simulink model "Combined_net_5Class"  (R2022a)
settings: Solver=FixedStepAuto  StartTime=0.0  StopTime=simtime  FixedStep=1  RelTol=1e-3
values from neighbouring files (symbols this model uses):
  simtime = length(SOC_CC{1, 1})    [Data_preparation.m]    (also in SimulationCycle.m = cell2mat(simtime_og(i)))
  SOH_predict = double(ans.SOHout(simtime))    [SimulationCycle.m]
undefined symbols (not defined in the file or in its folder): dSOC_mu_CC, dSOC_sig_CC, dv_mu_CC, dv_sig_CC, SOC_mu_CC, SOC_sig_CC, SOE_mu_CC, SOE_sig_CC
libraries: neural x183, deeplib x1
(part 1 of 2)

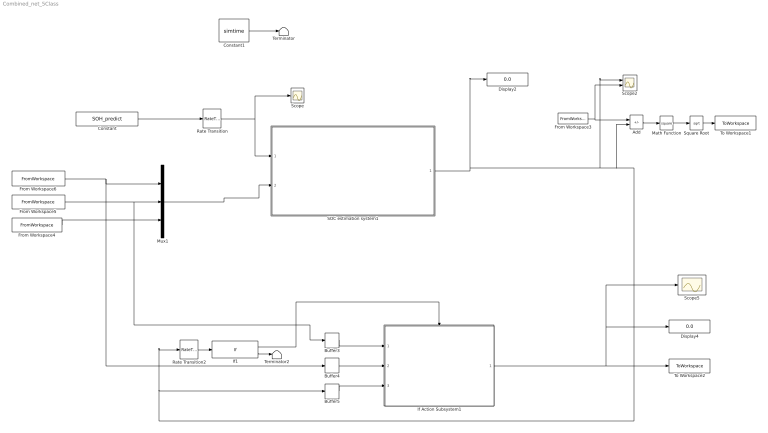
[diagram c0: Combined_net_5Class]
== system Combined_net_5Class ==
  Add : Sum  Inputs=+-
  Buffer3 : Buffer  N=120  OutputFrames=off
  Buffer4 : Buffer  N=120  OutputFrames=off
  Buffer5 : Buffer  N=120  OutputFrames=off
  Constant : Constant  Value=SOH_predict
  Constant1 : Constant  Value=simtime
  Display2 : Display
  Display4 : Display
  From Workspace3 : FromWorkspace  VariableName=SOC_GT
  From Workspace4 : FromWorkspace  VariableName=Temperature
  From Workspace5 : FromWorkspace  VariableName=Voltage  SampleTime=1
  From Workspace6 : FromWorkspace  VariableName=Current  SampleTime=1
  If Action Subsystem1 : Subsystem  TreatAsAtomicUnit=on
  If1 : If  IfExpression=u1 < 0.6
  Math Function : Math  Operator=square
  Mux1 : Mux  Inputs=3
  Rate Transition : RateTransition  OutPortSampleTime=1
  Rate Transition2 : RateTransition  OutPortSampleTime=1
  SOC estimation system1 : Subsystem
  Scope : Scope
  Scope2 : Scope  NumInputPorts=2
  Scope5 : Scope
  Square Root : Sqrt
  Terminator : Terminator
  Terminator2 : Terminator
  To Workspace1 : ToWorkspace  VariableName=SOC_abserror  SampleTime=-1
  To Workspace2 : ToWorkspace  VariableName=SOHout  SampleTime=-1
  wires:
  Rate Transition/1 -> Scope/1, SOC estimation system1/1(SOH)
  Buffer4/1 -> If Action Subsystem1/2(I)
  Buffer5/1 -> If Action Subsystem1/3(SOC)
  From Workspace6/1 -> Mux1/1, Buffer4/1
  Buffer3/1 -> If Action Subsystem1/1(V)
  From Workspace5/1 -> Buffer3/1, Mux1/2
  If1/1 -> If Action Subsystem1/Action
  If Action Subsystem1/1(Output) -> Scope5/1, Display4/1, To Workspace2/1
  Mux1/1 -> SOC estimation system1/2(Input)
  From Workspace4/1 -> Mux1/3
  If1/2 -> Terminator2/1
  Rate Transition2/1 -> If1/1
  Constant/1 -> Rate Transition/1
  Constant1/1 -> Terminator/1
  Math Function/1 -> Square Root/1
  From Workspace3/1 -> Add/1, Scope2/2
  Add/1 -> Math Function/1
  SOC estimation system1/1(SOC) -> Add/2, Rate Transition2/1, Buffer5/1, Scope2/1, Display2/1
  Square Root/1 -> To Workspace1/1

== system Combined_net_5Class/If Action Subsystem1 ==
  V : Inport
  I : Inport  Port=2
  SOC : Inport  Port=3
  Action Port : ActionPort  ActionPortLabel=if(u1 < 0.6)
  SOH estimation system : Subsystem
  Output : Outport
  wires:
  V/1 -> SOH estimation system/1(V)
  I/1 -> SOH estimation system/2(I)
  SOC/1 -> SOH estimation system/3(SOC)
  SOH estimation system/1(Input1) -> Output/1

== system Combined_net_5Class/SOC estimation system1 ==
  SOH : Inport
  Input : Inport  Port=2
  Class 1 : Subsystem
  Class 2 : Subsystem
  Class 3 : Subsystem
  Class 4 : Subsystem
  Class 5 : Subsystem
  If1 : If  IfExpression=0.96<u1  ElseIfExpressions=0.92<u1&u1<=0.96  ShowElse=off
  If2 : If  IfExpression=0.9<u1&u1<=0.92  ElseIfExpressions=0.87<u1&u1<=0.9  ShowElse=off
  If3 : If  IfExpression=u1<=0.87  ShowElse=off
  Merge1 : Merge  Inputs=5
  SOC : Outport
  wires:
  If3/1 -> Class 5/Action
  If2/2 -> Class 4/Action
  Class 3/1(SOC) -> Merge1/3
  Class 2/1(SOC) -> Merge1/2
  Class 1/1(SOC) -> Merge1/1
  If1/1 -> Class 1/Action
  Class 4/1(SOC) -> Merge1/4
  SOH/1 -> If3/1, If1/1, If2/1
  Class 5/1(SOC) -> Merge1/5
  Merge1/1 -> SOC/1
  If1/2 -> Class 2/Action
  If2/1 -> Class 3/Action
  Input/1 -> Class 1/1(Input), Class 2/1(Input1), Class 3/1(Input2), Class 4/1(Input), Class 5/1(Input)

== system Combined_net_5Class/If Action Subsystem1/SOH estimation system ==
  V : Inport
  I : Inport  Port=2
  SOC : Inport  Port=3
  Subsystem1 : Subsystem
  Subsystem2 : Subsystem
  Input1 : Outport
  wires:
  Subsystem1/4(SOE) -> Subsystem2/4(SOE)
  Subsystem1/1(dSOC) -> Subsystem2/1(dSOC)
  Subsystem1/2(dv) -> Subsystem2/2(dv)
  Subsystem1/3(SOC) -> Subsystem2/3(SOC)
  Subsystem2/1(Input1) -> Input1/1
  V/1 -> Subsystem1/1(V_03)
  I/1 -> Subsystem1/2(I_03)
  SOC/1 -> Subsystem1/3(SOC_03)

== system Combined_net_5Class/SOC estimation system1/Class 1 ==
  Input : Inport
  Action Port : ActionPort  ActionPortLabel=if(0.96<u1)
  Class 1 : Subsystem  mask{pi_input_1_delayed_1=[0.507169576059850246707583210081793367862701416015625;-0.46688362562526375398874733946286141872406005859375;-0.4863168465980416410587849895819090306758880615234375], ai_layer_2_delayed_1=-0.99999475321330122401519702179939486086368560791015625}
      mask prompts: pi_input_1_delayed_1 "Preprocessed initial input 1 state at timestep 0."; ai_layer_2_delayed_1 "Initial layer 2 state at timestep 0."
      mask help: NARX Neural Network
  SOC : Outport
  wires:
  Class 1/1(y) -> SOC/1
  Input/1 -> Class 1/1(x)

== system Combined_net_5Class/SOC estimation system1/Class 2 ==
  Input1 : Inport
  Action Port : ActionPort  ActionPortLabel=elseif(0.92<u1&u1<=0.96)
  Class 2 : Subsystem  mask{pi_input_1_delayed_1=[0.5002372291633718770498262529144994914531707763671875;-0.5901898734177215555263273927266709506511688232421875;-0.746840148698884487288296440965496003627777099609375], ai_layer_2_delayed_1=-0.99999334769130043820695163958589546382427215576171875}
      mask prompts: pi_input_1_delayed_1 "Preprocessed initial input 1 state at timestep 0."; ai_layer_2_delayed_1 "Initial layer 2 state at timestep 0."
      mask help: NARX Neural Network
  SOC : Outport
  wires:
  Input1/1 -> Class 2/1(x)
  Class 2/1(y) -> SOC/1

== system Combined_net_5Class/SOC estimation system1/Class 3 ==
  Input2 : Inport
  Action Port : ActionPort  ActionPortLabel=if(0.9<u1&u1<=0.92)
  Class 3 : Subsystem  mask{pi_input_1_delayed_1=[0.5070045647725482940160190992173738777637481689453125;-0.611404153034653230491812792024575173854827880859375;-1.455812101910827660589120569056831300258636474609375], ai_layer_2_delayed_1=-0.99999384932865742481311599476612173020839691162109375}
      mask prompts: pi_input_1_delayed_1 "Preprocessed initial input 1 state at timestep 0."; ai_layer_2_delayed_1 "Initial layer 2 state at timestep 0."
      mask help: NARX Neural Network
  SOC : Outport
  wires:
  Class 3/1(y) -> SOC/1
  Input2/1 -> Class 3/1(x)

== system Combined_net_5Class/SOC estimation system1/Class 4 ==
  Input : Inport
  Action Port : ActionPort  ActionPortLabel=elseif(0.87<u1&u1<=0.9)
  Class 4 : Subsystem  mask{pi_input_1_delayed_1=[0.5133640552995391015400628020870499312877655029296875;-0.60258438818565451811082311905920505523681640625;-0.865604575163398504145106926443986594676971435546875], ai_layer_2_delayed_1=-0.99999156111467002450154950565774925053119659423828125}
      mask prompts: pi_input_1_delayed_1 "Preprocessed initial input 1 state at timestep 0."; ai_layer_2_delayed_1 "Initial layer 2 state at timestep 0."
      mask help: NARX Neural Network
  SOC : Outport
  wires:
  Class 4/1(y) -> SOC/1
  Input/1 -> Class 4/1(x)

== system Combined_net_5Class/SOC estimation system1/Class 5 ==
  Input : Inport
  Action Port : ActionPort  ActionPortLabel=if(u1<=0.87)
  Class 5 : Subsystem  mask{pi_input_1_delayed_1=[0.521325559987726006028196934494189918041229248046875;-0.590428999869605064532152027823030948638916015625;-0.49791819740386955572830629535019397735595703125], ai_layer_2_delayed_1=-0.9999922448082632087107413099147379398345947265625}
      mask prompts: pi_input_1_delayed_1 "Preprocessed initial input 1 state at timestep 0."; ai_layer_2_delayed_1 "Initial layer 2 state at timestep 0."
      mask help: NARX Neural Network
  SOC : Outport
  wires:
  Class 5/1(y) -> SOC/1
  Input/1 -> Class 5/1(x)

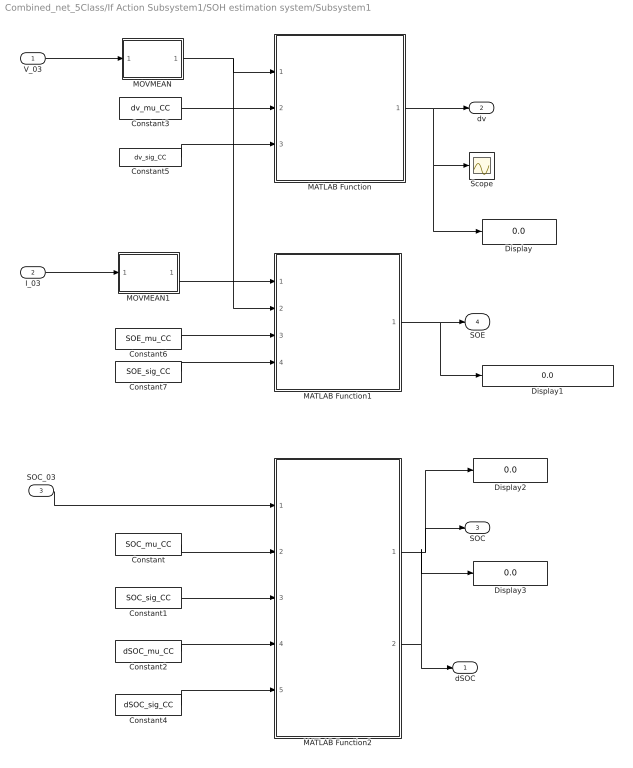
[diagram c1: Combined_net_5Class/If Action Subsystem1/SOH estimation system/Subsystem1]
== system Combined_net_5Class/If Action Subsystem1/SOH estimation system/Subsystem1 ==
  V_03 : Inport
  I_03 : Inport  Port=2
  SOC_03 : Inport  Port=3
  Constant : Constant  Value=SOC_mu_CC
  Constant1 : Constant  Value=SOC_sig_CC
  Constant2 : Constant  Value=dSOC_mu_CC
  Constant3 : Constant  Value=dv_mu_CC
  Constant4 : Constant  Value=dSOC_sig_CC
  Constant5 : Constant  Value=dv_sig_CC
  Constant6 : Constant  Value=SOE_mu_CC
  Constant7 : Constant  Value=SOE_sig_CC
  Display{,1..3} (4 alike) : Display
  MATLAB Function : MATLAB Function  TreatAsAtomicUnit=on
  MATLAB Function1 : MATLAB Function  TreatAsAtomicUnit=on
  MATLAB Function2 : MATLAB Function  TreatAsAtomicUnit=on
  MOVMEAN : MATLAB Function  TreatAsAtomicUnit=on
  MOVMEAN1 : MATLAB Function  TreatAsAtomicUnit=on
  Scope : Scope
  dSOC : Outport
  dv : Outport  Port=2
  SOC : Outport  Port=3
  SOE : Outport  Port=4
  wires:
  Constant4/1 -> MATLAB Function2/5(dSOC_sig_CC)
  Constant6/1 -> MATLAB Function1/3(SOE_mu_CC)
  Constant7/1 -> MATLAB Function1/4(SOE_sig_CC)
  Constant2/1 -> MATLAB Function2/4(dSOC_mu_CC)
  Constant5/1 -> MATLAB Function/3(dv_sig_CC)
  MATLAB Function2/2(dSOC) -> Display3/1, dSOC/1
  MATLAB Function/1(dV) -> Display/1, Scope/1, dv/1
  MATLAB Function2/1(SOC) -> Display2/1, SOC/1
  Constant3/1 -> MATLAB Function/2(dv_mu_CC)
  V_03/1 -> MOVMEAN/1(V)
  I_03/1 -> MOVMEAN1/1(I)
  Constant1/1 -> MATLAB Function2/3(SOC_sig_CC)
  Constant/1 -> MATLAB Function2/2(SOC_mu_CC)
  MATLAB Function1/1(SOE) -> Display1/1, SOE/1
  MOVMEAN/1(V_filt) -> MATLAB Function/1(V_03), MATLAB Function1/2(V_03)
  MOVMEAN1/1(I_filt) -> MATLAB Function1/1(I_03)
  SOC_03/1 -> MATLAB Function2/1(SOC_03)

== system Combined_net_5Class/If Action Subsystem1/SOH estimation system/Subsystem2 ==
  dSOC : Inport
  dv : Inport  Port=2
  SOC : Inport  Port=3
  SOE : Inport  Port=4
  Display : Display
  Mux2 : Mux
  Pulse Generator : DiscretePulseGenerator  PulseType=Time based  Period=120  PulseWidth=1/120*100  PhaseDelay=119
  Resettable Subsystem : Subsystem  TreatAsAtomicUnit=on
  Scope : Scope
  Input1 : Outport
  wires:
  Mux2/1 -> Display/1, Resettable Subsystem/2(Input1)
  dSOC/1 -> Mux2/1
  dv/1 -> Mux2/2
  SOC/1 -> Mux2/3
  SOE/1 -> Mux2/4
  Pulse Generator/1 -> Resettable Subsystem/1(Input), Resettable Subsystem/Reset, Scope/1
  Resettable Subsystem/1(Out1) -> Input1/1

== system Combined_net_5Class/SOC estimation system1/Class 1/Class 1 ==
  x : Inport  PortDimensions=3  SampleTime=1
  Layer 1 : Subsystem
  Layer 2 : Subsystem
  Process Input 1 : Subsystem
  Process Output 1 : Subsystem
  y : Outport  InitialOutput=0
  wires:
  x/1 -> Process Input 1/1(x)
  Process Output 1/1(y) -> y/1
  Process Input 1/1(p) -> Layer 1/1("p{1}")
  Layer 1/1("a{1}") -> [feedback1]
  [feedback1] -> Layer 2/1("a{1} ")
  Layer 2/1("a{2}") -> [feedback2], Process Output 1/1(a)
  [feedback2] -> Layer 1/2("a{2} ")

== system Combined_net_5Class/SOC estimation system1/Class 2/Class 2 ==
  x : Inport  PortDimensions=3  SampleTime=1
  Layer 1 : Subsystem
  Layer 2 : Subsystem
  Process Input 1 : Subsystem
  Process Output 1 : Subsystem
  y : Outport  InitialOutput=0
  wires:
  x/1 -> Process Input 1/1(x)
  Process Output 1/1(y) -> y/1
  Process Input 1/1(p) -> Layer 1/1("p{1}")
  Layer 1/1("a{1}") -> [feedback1]
  [feedback1] -> Layer 2/1("a{1} ")
  Layer 2/1("a{2}") -> [feedback2], Process Output 1/1(a)
  [feedback2] -> Layer 1/2("a{2} ")

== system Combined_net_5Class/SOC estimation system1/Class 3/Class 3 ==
  x : Inport  PortDimensions=3  SampleTime=1
  Layer 1 : Subsystem
  Layer 2 : Subsystem
  Process Input 1 : Subsystem
  Process Output 1 : Subsystem
  y : Outport  InitialOutput=0
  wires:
  x/1 -> Process Input 1/1(x)
  Process Output 1/1(y) -> y/1
  Process Input 1/1(p) -> Layer 1/1("p{1}")
  Layer 1/1("a{1}") -> [feedback1]
  [feedback1] -> Layer 2/1("a{1} ")
  Layer 2/1("a{2}") -> [feedback2], Process Output 1/1(a)
  [feedback2] -> Layer 1/2("a{2} ")

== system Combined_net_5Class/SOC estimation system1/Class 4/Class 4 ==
  x : Inport  PortDimensions=3  SampleTime=1
  Layer 1 : Subsystem
  Layer 2 : Subsystem
  Process Input 1 : Subsystem
  Process Output 1 : Subsystem
  y : Outport  InitialOutput=0
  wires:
  x/1 -> Process Input 1/1(x)
  Process Output 1/1(y) -> y/1
  Process Input 1/1(p) -> Layer 1/1("p{1}")
  Layer 1/1("a{1}") -> [feedback1]
  [feedback1] -> Layer 2/1("a{1} ")
  Layer 2/1("a{2}") -> [feedback2], Process Output 1/1(a)
  [feedback2] -> Layer 1/2("a{2} ")

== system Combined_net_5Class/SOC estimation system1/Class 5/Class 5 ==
  x : Inport  PortDimensions=3  SampleTime=1
  Layer 1 : Subsystem
  Layer 2 : Subsystem
  Process Input 1 : Subsystem
  Process Output 1 : Subsystem
  y : Outport  InitialOutput=0
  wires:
  x/1 -> Process Input 1/1(x)
  Process Output 1/1(y) -> y/1
  Process Input 1/1(p) -> Layer 1/1("p{1}")
  Layer 1/1("a{1}") -> [feedback1]
  [feedback1] -> Layer 2/1("a{1} ")
  Layer 2/1("a{2}") -> [feedback2], Process Output 1/1(a)
  [feedback2] -> Layer 1/2("a{2} ")

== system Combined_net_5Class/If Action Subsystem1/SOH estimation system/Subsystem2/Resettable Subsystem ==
  Input : Inport
  Input1 : Inport  Port=2
  Reset : ResetPort  DisableCoverage=on
  Triggered Subsystem : Subsystem  TreatAsAtomicUnit=on
  Out1 : Outport
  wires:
  Triggered Subsystem/1(Out1) -> Out1/1
  Input/1 -> Triggered Subsystem/Trigger
  Input1/1 -> Triggered Subsystem/1(u)

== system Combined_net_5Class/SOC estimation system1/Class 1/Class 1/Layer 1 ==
  "p{1}" : Inport  PortDimensions=3  SampleTime=1
  "a{2} " : Inport  Port=2  PortDimensions=1  SampleTime=1
  Delays 1 : Subsystem
  Delays 2 : Subsystem
  "IW{1,1}" : Subsystem
  "LW{1,2}" : Subsystem
  "b{1}" : Constant  Value=[2.34272603015963820638489778502844274044036865234375;-1.83098571478465554918102498049847781658172607421875;-0.79131154125893576889438918442465364933013916015625;-1.2076273263687624659468156096409074962139129638671875;0.84071386902655909079129514793748967349529266357421875;-0.53056878404548457606182410017936490476131439208984375;-0.0240383625943490740473063027593525475822389125823974609375;0.16604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
  netsum : Sum  Inputs=3  InputSameDT=on  SaturateOnIntegerOverflow=on
  tansig : neural/Transfer Functions/tansig
  "a{1}" : Outport  InitialOutput=[0;0;0;0;0;0;0;0;0;0;0;0;0;0;0]
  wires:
  "p{1}"/1 -> Delays 1/1("p{1}")
  Delays 1/1("pd{1,1}") -> "IW{1,1}"/1("pd{1,1}")
  "IW{1,1}"/1("iz{1,1}") -> netsum/1
  "a{2} "/1 -> Delays 2/1("p{1}")
  Delays 2/1("pd{1,2}") -> "LW{1,2}"/1("ad{1,2}")
  "LW{1,2}"/1("lz{1,2}") -> netsum/2
  "b{1}"/1 -> netsum/3
  netsum/1 -> tansig/1
  tansig/1 -> "a{1}"/1

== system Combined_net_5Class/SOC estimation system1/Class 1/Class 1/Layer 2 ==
  "a{1} " : Inport  PortDimensions=15  SampleTime=1
  Delays 1 : Subsystem
  "LW{2,1}" : Subsystem
  "b{2}" : Constant  Value=-0.2610570456976468722842810166184790432453155517578125
  netsum : Sum  Inputs=2  InputSameDT=on  SaturateOnIntegerOverflow=on
  purelin : neural/Transfer Functions/purelin
  "a{2}" : Outport  InitialOutput=0
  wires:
  "a{1} "/1 -> Delays 1/1("p{2}")
  Delays 1/1("pd{2,1}") -> "LW{2,1}"/1("ad{2,1}")
  "LW{2,1}"/1("lz{2,1}") -> netsum/1
  "b{2}"/1 -> netsum/2
  netsum/1 -> purelin/1
  purelin/1 -> "a{2}"/1

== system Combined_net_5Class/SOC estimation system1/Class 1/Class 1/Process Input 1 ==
  x : Inport  PortDimensions=3  SampleTime=1
  mapminmax : neural/Processing Functions/mapminmax  xmin=[-4.82500000000000017763568394003;2.50570000000000003836930773105;17.1380000000000016768808563938]  xmax=[1.5909999999999999698019337302;4.16500000000000003552713678801;25.1039999999999992041921359487]  ymin=-1  ymax=1
  p : Outport  PortDimensions=3  SampleTime=1
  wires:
  x/1 -> mapminmax/1
  mapminmax/1 -> p/1

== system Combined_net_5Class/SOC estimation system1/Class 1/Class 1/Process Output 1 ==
  a : Inport  PortDimensions=1  SampleTime=1
  mapminmax_reverse : neural/Processing Functions/mapminmax_reverse  xmin=-2.62341179120179950748424461959e-06  xmax=1.00000440635255594123975697585  ymin=-1  ymax=1
  y : Outport  PortDimensions=1  SampleTime=1
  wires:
  a/1 -> mapminmax_reverse/1
  mapminmax_reverse/1 -> y/1

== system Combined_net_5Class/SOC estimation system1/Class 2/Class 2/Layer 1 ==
  "p{1}" : Inport  PortDimensions=3  SampleTime=1
  "a{2} " : Inport  Port=2  PortDimensions=1  SampleTime=1
  Delays 1 : Subsystem
  Delays 2 : Subsystem
  "IW{1,1}" : Subsystem
  "LW{1,2}" : Subsystem
  "b{1}" : Constant  Value=[2.123679128509173619221428452874533832073211669921875;-2.87621199885181422217783619998954236507415771484375;-0.54420836494168567387674784185946919023990631103515625;-0.5394065908795988573132262899889610707759857177734375;0.85139936745729760669831875929958187043666839599609375;-1.1563643607811477931335275570745579898357391357421875;-0.61089692546734919442741329476120881736278533935546875;-0.197690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
  netsum : Sum  Inputs=3  InputSameDT=on  SaturateOnIntegerOverflow=on
  tansig : neural/Transfer Functions/tansig
  "a{1}" : Outport  InitialOutput=[0;0;0;0;0;0;0;0;0;0;0;0;0;0;0;0]
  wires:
  "p{1}"/1 -> Delays 1/1("p{1}")
  Delays 1/1("pd{1,1}") -> "IW{1,1}"/1("pd{1,1}")
  "IW{1,1}"/1("iz{1,1}") -> netsum/1
  "a{2} "/1 -> Delays 2/1("p{1}")
  Delays 2/1("pd{1,2}") -> "LW{1,2}"/1("ad{1,2}")
  "LW{1,2}"/1("lz{1,2}") -> netsum/2
  "b{1}"/1 -> netsum/3
  netsum/1 -> tansig/1
  tansig/1 -> "a{1}"/1

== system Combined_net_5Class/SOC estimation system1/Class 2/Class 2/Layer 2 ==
  "a{1} " : Inport  PortDimensions=16  SampleTime=1
  Delays 1 : Subsystem
  "LW{2,1}" : Subsystem
  "b{2}" : Constant  Value=0.1380564376019000061290853409445844590663909912109375
  netsum : Sum  Inputs=2  InputSameDT=on  SaturateOnIntegerOverflow=on
  purelin : neural/Transfer Functions/purelin
  "a{2}" : Outport  InitialOutput=0
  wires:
  "a{1} "/1 -> Delays 1/1("p{2}")
  Delays 1/1("pd{2,1}") -> "LW{2,1}"/1("ad{2,1}")
  "LW{2,1}"/1("lz{2,1}") -> netsum/1
  "b{2}"/1 -> netsum/2
  netsum/1 -> purelin/1
  purelin/1 -> "a{2}"/1

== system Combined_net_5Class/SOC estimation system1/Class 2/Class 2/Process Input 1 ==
  x : Inport  PortDimensions=3  SampleTime=1
  mapminmax : neural/Processing Functions/mapminmax  xmin=[-4.73300000000000054001247917768;2.63719999999999998863131622784;17.8219999999999991757704265183]  xmax=[1.59000000000000007993605777301;4.15399999999999991473487170879;28.5820000000000007389644451905]  ymin=-1  ymax=1
  p : Outport  PortDimensions=3  SampleTime=1
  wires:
  x/1 -> mapminmax/1
  mapminmax/1 -> p/1

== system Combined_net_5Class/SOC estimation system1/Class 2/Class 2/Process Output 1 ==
  a : Inport  PortDimensions=1  SampleTime=1
  mapminmax_reverse : neural/Processing Functions/mapminmax_reverse  xmin=-3.32617917940104848405083806662e-06  xmax=1.00000413879150817919594373961  ymin=-1  ymax=1
  y : Outport  PortDimensions=1  SampleTime=1
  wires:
  a/1 -> mapminmax_reverse/1
  mapminmax_reverse/1 -> y/1

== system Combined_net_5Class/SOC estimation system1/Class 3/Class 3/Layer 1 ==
  "p{1}" : Inport  PortDimensions=3  SampleTime=1
  "a{2} " : Inport  Port=2  PortDimensions=1  SampleTime=1
  Delays 1 : Subsystem
  Delays 2 : Subsystem
  "IW{1,1}" : Subsystem
  "LW{1,2}" : Subsystem
  "b{1}" : Constant  Value=[-1.93346371221756019309623297885991632938385009765625;1.7923652112547914239115698364912532269954681396484375;1.1238522489621971534035083095659501850605010986328125;0.323356733008480279334406759517150931060314178466796875;0.76493308526969572280762577065615914762020111083984375;-0.351089604850296443938617585445172153413295745849609375;0.33583797370279000471526842375169508159160614013671875;-0.46332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
  netsum : Sum  Inputs=3  InputSameDT=on  SaturateOnIntegerOverflow=on
  tansig : neural/Transfer Functions/tansig
  "a{1}" : Outport  InitialOutput=[0;0;0;0;0;0;0;0;0;0;0;0;0;0;0]
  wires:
  "p{1}"/1 -> Delays 1/1("p{1}")
  Delays 1/1("pd{1,1}") -> "IW{1,1}"/1("pd{1,1}")
  "IW{1,1}"/1("iz{1,1}") -> netsum/1
  "a{2} "/1 -> Delays 2/1("p{1}")
  Delays 2/1("pd{1,2}") -> "LW{1,2}"/1("ad{1,2}")
  "LW{1,2}"/1("lz{1,2}") -> netsum/2
  "b{1}"/1 -> netsum/3
  netsum/1 -> tansig/1
  tansig/1 -> "a{1}"/1

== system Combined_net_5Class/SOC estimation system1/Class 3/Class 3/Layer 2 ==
  "a{1} " : Inport  PortDimensions=15  SampleTime=1
  Delays 1 : Subsystem
  "LW{2,1}" : Subsystem
  "b{2}" : Constant  Value=0.272834520121191526076387390276067890226840972900390625
  netsum : Sum  Inputs=2  InputSameDT=on  SaturateOnIntegerOverflow=on
  purelin : neural/Transfer Functions/purelin
  "a{2}" : Outport  InitialOutput=0
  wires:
  "a{1} "/1 -> Delays 1/1("p{2}")
  Delays 1/1("pd{2,1}") -> "LW{2,1}"/1("ad{2,1}")
  "LW{2,1}"/1("lz{2,1}") -> netsum/1
  "b{2}"/1 -> netsum/2
  netsum/1 -> purelin/1
  purelin/1 -> "a{2}"/1

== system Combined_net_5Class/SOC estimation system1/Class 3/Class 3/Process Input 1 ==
  x : Inport  PortDimensions=3  SampleTime=1
  mapminmax : neural/Processing Functions/mapminmax  xmin=[-4.77700000000000013500311979442;2.6570000000000000284217094304;21.4740000000000001989519660128]  xmax=[1.57600000000000006750155989721;4.15470000000000005968558980385;31.5220000000000020179413695587]  ymin=-1  ymax=1
  p : Outport  PortDimensions=3  SampleTime=1
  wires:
  x/1 -> mapminmax/1
  mapminmax/1 -> p/1

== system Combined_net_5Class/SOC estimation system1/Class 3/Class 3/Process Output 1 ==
  a : Inport  PortDimensions=1  SampleTime=1
  mapminmax_reverse : neural/Processing Functions/mapminmax_reverse  xmin=-3.07535918984610110574521267546e-06  xmax=1.00000457212472371182343522378  ymin=-1  ymax=1
  y : Outport  PortDimensions=1  SampleTime=1
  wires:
  a/1 -> mapminmax_reverse/1
  mapminmax_reverse/1 -> y/1

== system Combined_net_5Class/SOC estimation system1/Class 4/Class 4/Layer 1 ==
  "p{1}" : Inport  PortDimensions=3  SampleTime=1
  "a{2} " : Inport  Port=2  PortDimensions=1  SampleTime=1
  Delays 1 : Subsystem
  Delays 2 : Subsystem
  "IW{1,1}" : Subsystem
  "LW{1,2}" : Subsystem
  "b{1}" : Constant  Value=[-2.688444044962437828871770761907100677490234375;0.858381113224772729353162503684870898723602294921875;-2.222715747204785596835563410422764718532562255859375;1.3209762857863693863436083120177499949932098388671875;-0.8915787953875426996575015436974354088306427001953125;-0.88615966223780884281069347707671113312244415283203125;0.280218393721010927688297442728071473538875579833984375;0.21524348971530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
  netsum : Sum  Inputs=3  InputSameDT=on  SaturateOnIntegerOverflow=on
  tansig : neural/Transfer Functions/tansig
  "a{1}" : Outport  InitialOutput=[0;0;0;0;0;0;0;0;0;0;0;0;0;0;0]
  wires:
  "p{1}"/1 -> Delays 1/1("p{1}")
  Delays 1/1("pd{1,1}") -> "IW{1,1}"/1("pd{1,1}")
  "IW{1,1}"/1("iz{1,1}") -> netsum/1
  "a{2} "/1 -> Delays 2/1("p{1}")
  Delays 2/1("pd{1,2}") -> "LW{1,2}"/1("ad{1,2}")
  "LW{1,2}"/1("lz{1,2}") -> netsum/2
  "b{1}"/1 -> netsum/3
  netsum/1 -> tansig/1
  tansig/1 -> "a{1}"/1

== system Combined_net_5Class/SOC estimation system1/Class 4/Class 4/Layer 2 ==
  "a{1} " : Inport  PortDimensions=15  SampleTime=1
  Delays 1 : Subsystem
  "LW{2,1}" : Subsystem
  "b{2}" : Constant  Value=0.045626078950611735629561138694043620489537715911865234375
  netsum : Sum  Inputs=2  InputSameDT=on  SaturateOnIntegerOverflow=on
  purelin : neural/Transfer Functions/purelin
  "a{2}" : Outport  InitialOutput=0
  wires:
  "a{1} "/1 -> Delays 1/1("p{2}")
  Delays 1/1("pd{2,1}") -> "LW{2,1}"/1("ad{2,1}")
  "LW{2,1}"/1("lz{2,1}") -> netsum/1
  "b{2}"/1 -> netsum/2
  netsum/1 -> purelin/1
  purelin/1 -> "a{2}"/1

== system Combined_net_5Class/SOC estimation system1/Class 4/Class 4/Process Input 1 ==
  x : Inport  PortDimensions=3  SampleTime=1
  mapminmax : neural/Processing Functions/mapminmax  xmin=[-4.91600000000000036948222259525;2.64660000000000028563817977556;18.5259999999999998010480339872]  xmax=[1.59400000000000008348877145181;4.16340000000000021174173525651;28.3180000000000013926637620898]  ymin=-1  ymax=1
  p : Outport  PortDimensions=3  SampleTime=1
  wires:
  x/1 -> mapminmax/1
  mapminmax/1 -> p/1

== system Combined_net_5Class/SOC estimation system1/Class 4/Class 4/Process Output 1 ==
  a : Inport  PortDimensions=1  SampleTime=1
  mapminmax_reverse : neural/Processing Functions/mapminmax_reverse  xmin=-4.21949321457851519659313158095e-06  xmax=1.00000776066564278643511443079  ymin=-1  ymax=1
  y : Outport  PortDimensions=1  SampleTime=1
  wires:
  a/1 -> mapminmax_reverse/1
  mapminmax_reverse/1 -> y/1

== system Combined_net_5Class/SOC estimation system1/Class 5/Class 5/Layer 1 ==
  "p{1}" : Inport  PortDimensions=3  SampleTime=1
  "a{2} " : Inport  Port=2  PortDimensions=1  SampleTime=1
  Delays 1 : Subsystem
  Delays 2 : Subsystem
  "IW{1,1}" : Subsystem
  "LW{1,2}" : Subsystem
  "b{1}" : Constant  Value=[-1.9239326886795684590225619103875942528247833251953125;-1.4156259333430829538968964698142372071743011474609375;-1.8809744346361843003734293233719654381275177001953125;-1.106968201899322767900457620271481573581695556640625;1.16695809702027997190043606678955256938934326171875;1.0579085603689832861817876619170419871807098388671875;0.33221840417104486764543480603606440126895904541015625;-0.035398306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
  netsum : Sum  Inputs=3  InputSameDT=on  SaturateOnIntegerOverflow=on
  tansig : neural/Transfer Functions/tansig
  "a{1}" : Outport  InitialOutput=[0;0;0;0;0;0;0;0;0;0;0;0;0;0;0;0;0;0]
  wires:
  "p{1}"/1 -> Delays 1/1("p{1}")
  Delays 1/1("pd{1,1}") -> "IW{1,1}"/1("pd{1,1}")
  "IW{1,1}"/1("iz{1,1}") -> netsum/1
  "a{2} "/1 -> Delays 2/1("p{1}")
  Delays 2/1("pd{1,2}") -> "LW{1,2}"/1("ad{1,2}")
  "LW{1,2}"/1("lz{1,2}") -> netsum/2
  "b{1}"/1 -> netsum/3
  netsum/1 -> tansig/1
  tansig/1 -> "a{1}"/1

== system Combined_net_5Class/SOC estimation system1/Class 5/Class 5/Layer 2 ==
  "a{1} " : Inport  PortDimensions=18  SampleTime=1
  Delays 1 : Subsystem
  "LW{2,1}" : Subsystem
  "b{2}" : Constant  Value=0.2439901834476533026840883167096762917935848236083984375
  netsum : Sum  Inputs=2  InputSameDT=on  SaturateOnIntegerOverflow=on
  purelin : neural/Transfer Functions/purelin
  "a{2}" : Outport  InitialOutput=0
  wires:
  "a{1} "/1 -> Delays 1/1("p{2}")
  Delays 1/1("pd{2,1}") -> "LW{2,1}"/1("ad{2,1}")
  "LW{2,1}"/1("lz{2,1}") -> netsum/1
  "b{2}"/1 -> netsum/2
  netsum/1 -> purelin/1
  purelin/1 -> "a{2}"/1

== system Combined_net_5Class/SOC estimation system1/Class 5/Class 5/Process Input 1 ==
  x : Inport  PortDimensions=3  SampleTime=1
  mapminmax : neural/Processing Functions/mapminmax  xmin=[-4.94800000000000039790393202566;2.6339000000000001300293206441;17.1340000000000003410605131648]  xmax=[1.57000000000000006217248937901;4.16769999999999996020960679743;25.3000000000000007105427357601]  ymin=-1  ymax=1
  p : Outport  PortDimensions=3  SampleTime=1
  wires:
  x/1 -> mapminmax/1
  mapminmax/1 -> p/1

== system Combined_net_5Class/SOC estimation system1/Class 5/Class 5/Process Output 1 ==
  a : Inport  PortDimensions=1  SampleTime=1
  mapminmax_reverse : neural/Processing Functions/mapminmax_reverse  xmin=-3.87764264893447179729721319141e-06  xmax=1.0000081866738852465203990505  ymin=-1  ymax=1
  y : Outport  PortDimensions=1  SampleTime=1
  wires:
  a/1 -> mapminmax_reverse/1
  mapminmax_reverse/1 -> y/1

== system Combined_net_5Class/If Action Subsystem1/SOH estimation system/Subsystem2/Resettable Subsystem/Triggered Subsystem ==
  u : Inport
  Trigger : TriggerPort  TriggerType=falling  VariantControl=(inherit)
  Display : Display
  Scope : Scope
  Stateful Predict : deeplib/Stateful Predict  Network=Network from MAT-file  NetworkFunction=untitled  NetworkFilePath=E:\Thesis\Conclusion step\net.mat  InputDataFormats={ '', '' }  SampleTime=-1  ForceInterpretedSim=off  EnableDLNetwork=on
  Out1 : Outport
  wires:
  u/1 -> Stateful Predict/1, Scope/1, Display/1
  Stateful Predict/1 -> Out1/1

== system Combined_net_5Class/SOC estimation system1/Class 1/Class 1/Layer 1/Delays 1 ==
  "p{1}" : Inport  PortDimensions=3  SampleTime=1
  Delay 1 : UnitDelay  InitialCondition=pi_input_1_delayed_1
  mux : Mux  Inputs=2
  "pd{1,1}" : Outport
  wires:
  "p{1}"/1 -> Delay 1/1, mux/1
  Delay 1/1 -> mux/2
  mux/1 -> "pd{1,1}"/1

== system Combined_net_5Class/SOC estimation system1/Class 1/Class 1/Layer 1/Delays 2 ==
  "p{1}" : Inport  PortDimensions=1  SampleTime=1
  Delay 1 : UnitDelay  InitialCondition=ai_layer_2_delayed_1
  mux : Mux  Inputs=1
  "pd{1,2}" : Outport
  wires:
  "p{1}"/1 -> Delay 1/1
  Delay 1/1 -> mux/1
  mux/1 -> "pd{1,2}"/1

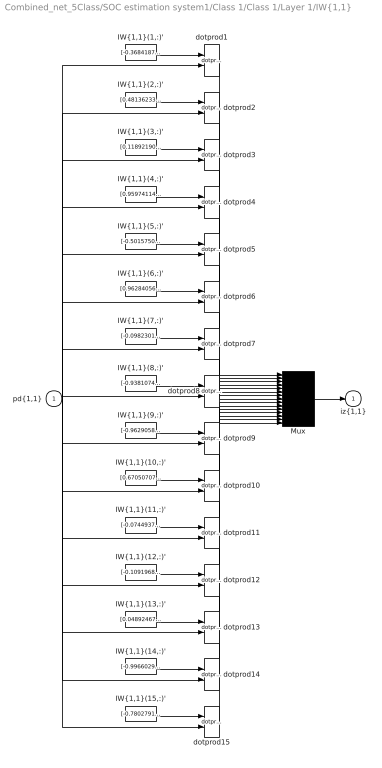
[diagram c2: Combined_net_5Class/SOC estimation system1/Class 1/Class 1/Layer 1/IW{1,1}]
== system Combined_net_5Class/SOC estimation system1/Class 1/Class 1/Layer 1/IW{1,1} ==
  "pd{1,1}" : Inport  PortDimensions=6  SampleTime=1
  "IW{1,1}(1,:)'" : Constant  Value=[-0.36841871672555603911547450479702092707157135009765625;0.95481863811988365586813642948982305824756622314453125;0.226878529936702599822950787711306475102901458740234375;0.036258766201381888161225930389264249242842197418212890625;0.3238678699587700382522825748310424387454986572265625;-0.84200791510325945221637766735511831939220428466796875]
  "IW{1,1}(10,:)'" : Constant  Value=[0.67050707720070523709665621936437673866748809814453125;0.882956797146274841026070134830661118030548095703125;-0.90123173513004661838721176536637358367443084716796875;0.89515060785826994216307639362639747560024261474609375;-0.805115591223422466526926655205897986888885498046875;-0.2593277792147092863928037331788800656795501708984375]
  "IW{1,1}(11,:)'" : Constant  Value=[-0.0744937388110009646169373809243552386760711669921875;0.91481150331324145863476360318600200116634368896484375;-0.0033589550935993598736184484465638888650573790073394775390625;0.09387686590177278522784121150834835134446620941162109375;-0.99451251190708223059999681936460547149181365966796875;-0.0003307952570151217433665202793946491510723717510700225830078125]
  "IW{1,1}(12,:)'" : Constant  Value=[-0.10919681936643919895058019164935103617608547210693359375;0.50465640273350442779332070131204091012477874755859375;0.00167935474555881941553792113808185604284517467021942138671875;0.090898075716160431358758842179668135941028594970703125;-0.421892519785072861449037873171619139611721038818359375;0.004083310809217589355812894069686080911196768283843994140625]
  "IW{1,1}(13,:)'" : Constant  Value=[0.048924672243263016280234722898967447690665721893310546875;-0.53987449057316327927225074745365418493747711181640625;0.00170226104659932341023331758833592175506055355072021484375;-0.058328940083118230308656393390265293419361114501953125;0.57776802472895305573530322362785227596759796142578125;-0.00015032127929270978146554516019506309021380729973316192626953125]
  "IW{1,1}(14,:)'" : Constant  Value=[-0.99660291683138291229937522075488232076168060302734375;0.5911312952433938061602702873642556369304656982421875;1.14540739846979366944879075163044035434722900390625;-0.3381076514679877131897001163451932370662689208984375;0.45894832786268346946911833583726547658443450927734375;-0.70176558995015925201954587464570067822933197021484375]
  "IW{1,1}(15,:)'" : Constant  Value=[-0.7802791008156886309876654195250011980533599853515625;1.0534129951958177695559015774051658809185028076171875;-0.03448938205268679835224787666447809897363185882568359375;0.94691798651251091190061970337410457432270050048828125;0.0231481724065754346231216231899452395737171173095703125;-0.5027468755563602176295034951181150972843170166015625]
  "IW{1,1}(2,:)'" : Constant  Value=[0.481362338278815193870485700244898907840251922607421875;-1.50652710762162467261759957182221114635467529296875;-0.2359262305730511488643941220288979820907115936279296875;-0.1406423235510661229330509058854659087955951690673828125;0.1819515858690983478584968224822659976780414581298828125;0.86381133633920403891437445054179988801479339599609375]
  "IW{1,1}(3,:)'" : Constant  Value=[0.11892190500532838492997456114608212374150753021240234375;-0.24493184734591633144873412675224244594573974609375;-0.00451567345059881997126893793392810039222240447998046875;-0.08059998953516155084653149742734967730939388275146484375;0.07911717353434512267629230564125464297831058502197265625;-0.00710306128001607188504618051183570059947669506072998046875]
  "IW{1,1}(4,:)'" : Constant  Value=[0.95974114664550247422170059508061967790126800537109375;-0.8796676994389194259582609447534196078777313232421875;0.9728248784750912481200657566660083830356597900390625;-0.70361057504988477884211306445649825036525726318359375;0.6194834636783788095470981716061942279338836669921875;0.61913161067906596901622151563060469925403594970703125]
  "IW{1,1}(5,:)'" : Constant  Value=[-0.50157500574550883953861557529307901859283447265625;-0.375530160518852185180804781339247711002826690673828125;0.01501545548960662480875161151061547570861876010894775390625;0.757425535532789684367571680922992527484893798828125;-0.77182219089220105434634433549945242702960968017578125;-0.0759994756633779744436907321869512088596820831298828125]
  "IW{1,1}(6,:)'" : Constant  Value=[0.9628405697273880736730689022806473076343536376953125;-0.632510343955252185565996114746667444705963134765625;0.35396101720878470064945986450766213238239288330078125;-0.60680374926630076259925772319547832012176513671875;0.177448918867727456483152082000742666423320770263671875;0.9817426047833206492754243299714289605617523193359375]
  "IW{1,1}(7,:)'" : Constant  Value=[-0.09823010496840246796868001410985016264021396636962890625;-1.185310142409820688413901734747923910617828369140625;0.1908758613743539445106733865031856112182140350341796875;-1.1914761953630537139048328754142858088016510009765625;0.39827398536536140483121926081366837024688720703125;0.90973345961705021078813615531544201076030731201171875]
  "IW{1,1}(8,:)'" : Constant  Value=[-0.93810741037665390518185404289397411048412322998046875;-1.2595077433783707920866845597629435360431671142578125;-0.78652190025548751606265795999206602573394775390625;-0.7895482370616810907648641659761779010295867919921875;0.24445192827118944478570483624935150146484375;0.34046059489771918205036627114168368279933929443359375]
  "IW{1,1}(9,:)'" : Constant  Value=[-0.962905875728648386058239339035935699939727783203125;-0.99822741054854535747153931879438459873199462890625;1.4514584750111370059499904527910985052585601806640625;-0.338753693920172793685452461431850679218769073486328125;-0.2495656714555981314784816049723303876817226409912109375;-0.0823827548058631842220478347371681593358516693115234375]
  Mux : Mux  Inputs=15
  dotprod{1..15} (15 alike) : neural/Weight Functions/dotprod
  "iz{1,1}" : Outport
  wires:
  "IW{1,1}(1,:)'"/1 -> dotprod1/1
  "pd{1,1}"/1 -> dotprod1/2, dotprod2/2, dotprod3/2, dotprod4/2, dotprod5/2, dotprod6/2, dotprod7/2, dotprod8/2, dotprod9/2, dotprod10/2, dotprod11/2, dotprod12/2, dotprod13/2, dotprod14/2, dotprod15/2
  dotprod1/1 -> Mux/1
  "IW{1,1}(2,:)'"/1 -> dotprod2/1
  dotprod2/1 -> Mux/2
  "IW{1,1}(3,:)'"/1 -> dotprod3/1
  dotprod3/1 -> Mux/3
  "IW{1,1}(4,:)'"/1 -> dotprod4/1
  dotprod4/1 -> Mux/4
  "IW{1,1}(5,:)'"/1 -> dotprod5/1
  dotprod5/1 -> Mux/5
  "IW{1,1}(6,:)'"/1 -> dotprod6/1
  dotprod6/1 -> Mux/6
  "IW{1,1}(7,:)'"/1 -> dotprod7/1
  dotprod7/1 -> Mux/7
  "IW{1,1}(8,:)'"/1 -> dotprod8/1
  dotprod8/1 -> Mux/8
  "IW{1,1}(9,:)'"/1 -> dotprod9/1
  dotprod9/1 -> Mux/9
  "IW{1,1}(10,:)'"/1 -> dotprod10/1
  dotprod10/1 -> Mux/10
  "IW{1,1}(11,:)'"/1 -> dotprod11/1
  dotprod11/1 -> Mux/11
  "IW{1,1}(12,:)'"/1 -> dotprod12/1
  dotprod12/1 -> Mux/12
  "IW{1,1}(13,:)'"/1 -> dotprod13/1
  dotprod13/1 -> Mux/13
  "IW{1,1}(14,:)'"/1 -> dotprod14/1
  dotprod14/1 -> Mux/14
  "IW{1,1}(15,:)'"/1 -> dotprod15/1
  dotprod15/1 -> Mux/15
  Mux/1 -> "iz{1,1}"/1

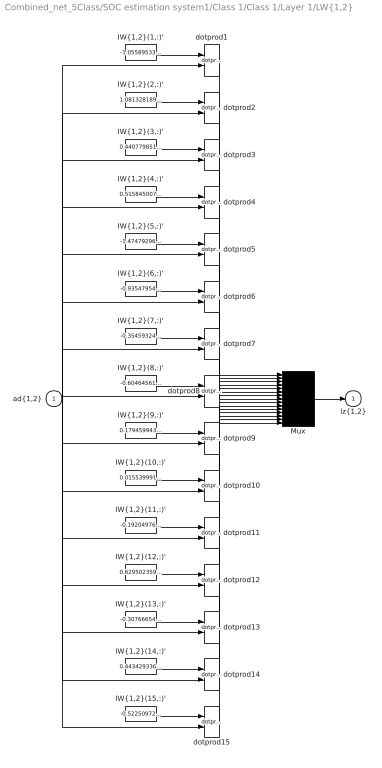
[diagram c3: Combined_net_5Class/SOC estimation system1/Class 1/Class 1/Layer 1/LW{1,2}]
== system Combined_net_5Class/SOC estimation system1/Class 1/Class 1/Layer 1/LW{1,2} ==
  "ad{1,2}" : Inport  PortDimensions=1  SampleTime=1
  "IW{1,2}(1,:)'" : Constant  Value=-1.0558953399790829141835502014146186411380767822265625
  "IW{1,2}(10,:)'" : Constant  Value=0.0155399911340668960002542320353313698433339595794677734375
  "IW{1,2}(11,:)'" : Constant  Value=-0.1920497660372149917318296274970634840428829193115234375
  "IW{1,2}(12,:)'" : Constant  Value=0.62950235962305978176800635992549359798431396484375
  "IW{1,2}(13,:)'" : Constant  Value=-0.30766654353943623245726257664500735700130462646484375
  "IW{1,2}(14,:)'" : Constant  Value=0.443429336021788522703701573846046812832355499267578125
  "IW{1,2}(15,:)'" : Constant  Value=-0.52250972552172625373856362784863449633121490478515625
  "IW{1,2}(2,:)'" : Constant  Value=1.08132818981622680354348631226457655429840087890625
  "IW{1,2}(3,:)'" : Constant  Value=0.440779851117324483755766095782746560871601104736328125
  "IW{1,2}(4,:)'" : Constant  Value=0.51584500712902159325068396356073208153247833251953125
  "IW{1,2}(5,:)'" : Constant  Value=-1.47479296662152048469351939274929463863372802734375
  "IW{1,2}(6,:)'" : Constant  Value=-0.935479542831488597443012622534297406673431396484375
  "IW{1,2}(7,:)'" : Constant  Value=-0.354593245240020948916281895435531623661518096923828125
  "IW{1,2}(8,:)'" : Constant  Value=-0.6046456148812133779557598245446570217609405517578125
  "IW{1,2}(9,:)'" : Constant  Value=0.1794599438126181223385202656572801060974597930908203125
  Mux : Mux  Inputs=15
  dotprod{1..15} (15 alike) : neural/Weight Functions/dotprod
  "lz{1,2}" : Outport
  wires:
  "IW{1,2}(1,:)'"/1 -> dotprod1/1
  "ad{1,2}"/1 -> dotprod1/2, dotprod2/2, dotprod3/2, dotprod4/2, dotprod5/2, dotprod6/2, dotprod7/2, dotprod8/2, dotprod9/2, dotprod10/2, dotprod11/2, dotprod12/2, dotprod13/2, dotprod14/2, dotprod15/2
  dotprod1/1 -> Mux/1
  "IW{1,2}(2,:)'"/1 -> dotprod2/1
  dotprod2/1 -> Mux/2
  "IW{1,2}(3,:)'"/1 -> dotprod3/1
  dotprod3/1 -> Mux/3
  "IW{1,2}(4,:)'"/1 -> dotprod4/1
  dotprod4/1 -> Mux/4
  "IW{1,2}(5,:)'"/1 -> dotprod5/1
  dotprod5/1 -> Mux/5
  "IW{1,2}(6,:)'"/1 -> dotprod6/1
  dotprod6/1 -> Mux/6
  "IW{1,2}(7,:)'"/1 -> dotprod7/1
  dotprod7/1 -> Mux/7
  "IW{1,2}(8,:)'"/1 -> dotprod8/1
  dotprod8/1 -> Mux/8
  "IW{1,2}(9,:)'"/1 -> dotprod9/1
  dotprod9/1 -> Mux/9
  "IW{1,2}(10,:)'"/1 -> dotprod10/1
  dotprod10/1 -> Mux/10
  "IW{1,2}(11,:)'"/1 -> dotprod11/1
  dotprod11/1 -> Mux/11
  "IW{1,2}(12,:)'"/1 -> dotprod12/1
  dotprod12/1 -> Mux/12
  "IW{1,2}(13,:)'"/1 -> dotprod13/1
  dotprod13/1 -> Mux/13
  "IW{1,2}(14,:)'"/1 -> dotprod14/1
  dotprod14/1 -> Mux/14
  "IW{1,2}(15,:)'"/1 -> dotprod15/1
  dotprod15/1 -> Mux/15
  Mux/1 -> "lz{1,2}"/1

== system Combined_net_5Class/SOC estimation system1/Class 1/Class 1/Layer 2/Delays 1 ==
  "p{2}" : Inport  PortDimensions=15  SampleTime=1
  mux : Mux  Inputs=1
  "pd{2,1}" : Outport
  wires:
  "p{2}"/1 -> mux/1
  mux/1 -> "pd{2,1}"/1

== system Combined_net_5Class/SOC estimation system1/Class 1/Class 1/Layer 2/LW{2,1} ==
  "ad{2,1}" : Inport  PortDimensions=15  SampleTime=1
  "IW{2,1}(1,:)'" : Constant  Value=[-0.4054339128384827350970454062917269766330718994140625;-0.150291660026959761342624233293463476002216339111328125;0.399718217310838286326912793811061419546604156494140625;3.55968054837466467703495365260124572159838862717151641845703125e-05;-0.0023970249922561893095307450352038358687423169612884521484375;-0.000111633850285505030063178122379241585804265923798084259033203125;-8.764101469894136078268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
  Mux : Mux  Inputs=1
  dotprod1 : neural/Weight Functions/dotprod
  "lz{2,1}" : Outport
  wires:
  "IW{2,1}(1,:)'"/1 -> dotprod1/1
  "ad{2,1}"/1 -> dotprod1/2
  dotprod1/1 -> Mux/1
  Mux/1 -> "lz{2,1}"/1

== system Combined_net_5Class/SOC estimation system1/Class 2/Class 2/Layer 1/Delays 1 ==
  "p{1}" : Inport  PortDimensions=3  SampleTime=1
  Delay 1 : UnitDelay  InitialCondition=pi_input_1_delayed_1
  mux : Mux  Inputs=2
  "pd{1,1}" : Outport
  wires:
  "p{1}"/1 -> Delay 1/1, mux/1
  Delay 1/1 -> mux/2
  mux/1 -> "pd{1,1}"/1

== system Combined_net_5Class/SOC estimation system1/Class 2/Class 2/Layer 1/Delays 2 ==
  "p{1}" : Inport  PortDimensions=1  SampleTime=1
  Delay 1 : UnitDelay  InitialCondition=ai_layer_2_delayed_1
  mux : Mux  Inputs=1
  "pd{1,2}" : Outport
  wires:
  "p{1}"/1 -> Delay 1/1
  Delay 1/1 -> mux/1
  mux/1 -> "pd{1,2}"/1

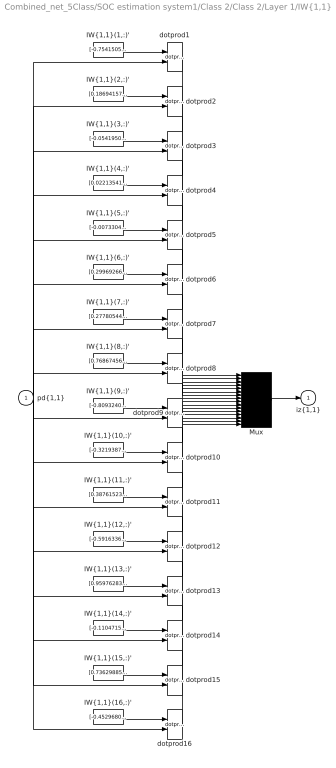
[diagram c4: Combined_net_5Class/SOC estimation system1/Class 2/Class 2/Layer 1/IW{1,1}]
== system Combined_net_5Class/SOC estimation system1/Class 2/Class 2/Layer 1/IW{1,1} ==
  "pd{1,1}" : Inport  PortDimensions=6  SampleTime=1
  "IW{1,1}(1,:)'" : Constant  Value=[-0.75415057701016630087309522423311136662960052490234375;-1.0602445863909493173338205451727844774723052978515625;-0.403611403758913578343481276533566415309906005859375;-0.042370088051090014358290858353939256630837917327880859375;-0.358462732167448228093320494735962711274623870849609375;0.19714157803441978433767189926584251224994659423828125]
  "IW{1,1}(10,:)'" : Constant  Value=[-0.321938743765563140097896166480495594441890716552734375;-0.368191606853078778893717526443651877343654632568359375;0.185129768716035203457437319229939021170139312744140625;0.2043650302890716308201746187478420324623584747314453125;0.8826891966589267557452558321529068052768707275390625;-0.1839543464343567913399368762839003466069698333740234375]
  "IW{1,1}(11,:)'" : Constant  Value=[0.387615236096453485981072617505560629069805145263671875;0.196254128563643603921917701882193796336650848388671875;-0.276725361207262654517080591176636517047882080078125;-0.257025784530381440351476385330897755920886993408203125;-0.64905830459941571408677418730803765356540679931640625;0.2744228849555911953217446352937258780002593994140625]
  "IW{1,1}(12,:)'" : Constant  Value=[-0.5916336524327923118704575244919396936893463134765625;0.85700047195421646950563854261417873203754425048828125;-0.2404315479020745771610023666653432883322238922119140625;-0.28768874058510063296267844634712673723697662353515625;-0.99971847270303026977700255883974023163318634033203125;1.2210817816879375730110268705175258219242095947265625]
  "IW{1,1}(13,:)'" : Constant  Value=[0.9597628331124570255639127935864962637424468994140625;-0.88562204242495046191407936930772848427295684814453125;-0.1760286219065132773398119070407119579613208770751953125;0.0927457879735908985452397246262989938259124755859375;0.722615388006634606909983631339855492115020751953125;-0.6131752174861262449923060557921417057514190673828125]
  "IW{1,1}(14,:)'" : Constant  Value=[-0.110471583141628804103362426758394576609134674072265625;0.74354882610338679516104321010061539709568023681640625;1.03451333545073875797015716671012341976165771484375;-0.3431922329775043412070090198540128767490386962890625;0.39852851406454170568594008727814070880413055419921875;1.0966067477081173908715072684572078287601470947265625]
  "IW{1,1}(15,:)'" : Constant  Value=[0.736298859452847676010378563660196959972381591796875;0.2927685967548416812178402324207127094268798828125;0.51499227548445725144432572051300667226314544677734375;-0.62644998419346598073076393120572902262210845947265625;0.923259144993893610120494486181996762752532958984375;-1.3496213250437367747736061573959887027740478515625]
  "IW{1,1}(16,:)'" : Constant  Value=[-0.452968098562966658970907474213163368403911590576171875;0.60195997671845280496683017190662212669849395751953125;1.244737450531746336679361775168217718601226806640625;-0.267275168753866976256716725401929579675197601318359375;-0.79176482905028933156899029199848882853984832763671875;-0.373843491362180591064401369294500909745693206787109375]
  "IW{1,1}(2,:)'" : Constant  Value=[0.1869415714832383390575643034026143141090869903564453125;-0.6690372979258658592272013265755958855152130126953125;0.012759415210163493892281394437304697930812835693359375;-0.1072554799884200826820546126327826641499996185302734375;0.89086845426267691205879373228526674211025238037109375;0.0110784479353181752880885824197321198880672454833984375]
  "IW{1,1}(3,:)'" : Constant  Value=[-0.054195072472333072344241600148961879312992095947265625;0.6470127629050310691383174344082362949848175048828125;0.02958524062784954888893906854718807153403759002685546875;0.0496634210674790910200471216739970259368419647216796875;-0.6458067868671537592462073007482104003429412841796875;-0.02986473920004327486932282909037894569337368011474609375]
  "IW{1,1}(4,:)'" : Constant  Value=[0.02213541632722655638776387831967440433800220489501953125;-0.240899083486367349138390636653639376163482666015625;-0.01191506308611154328624959219951051636599004268646240234375;-0.0199166550633538379233566928405707585625350475311279296875;0.239544708041063703074513568935799412429332733154296875;0.01207602017044143334623118590798185323365032672882080078125]
  "IW{1,1}(5,:)'" : Constant  Value=[-0.00733044418628346627908598520662053488194942474365234375;-0.0084764079610155744493038554310260224156081676483154296875;0.00490719146096560941694431079440619214437901973724365234375;0.004677380583939102880186577948506965185515582561492919921875;0.017297844939912286610361746852504438720643520355224609375;-0.004879080304036523436927996755230196868069469928741455078125]
  "IW{1,1}(6,:)'" : Constant  Value=[0.299692666422208875420807316913851536810398101806640625;-0.68961822746760048641334606145392172038555145263671875;0.7974891197889293348310957298963330686092376708984375;-1.4092010466297455462125753911095671355724334716796875;0.304297230825261666442571595325716771185398101806640625;0.457098009382508274622836097478284500539302825927734375]
  "IW{1,1}(7,:)'" : Constant  Value=[0.27780544103598447946978922118432819843292236328125;-1.1700995366539628239621606553555466234683990478515625;-0.63772016572320489036229673729394562542438507080078125;-0.9373334711565082244533186894841492176055908203125;-0.89278078863036325341084875617525540292263031005859375;0.5381445509060254206445961244753561913967132568359375]
  "IW{1,1}(8,:)'" : Constant  Value=[0.7686745628797455598402166287996806204319000244140625;0.90511933117887710675830703621613793075084686279296875;-0.4936655679901107429685680472175590693950653076171875;0.62958244947628572152353854107786901295185089111328125;0.8431080009011642228955452083027921617031097412109375;-0.7162116048413749158640939640463329851627349853515625]
  "IW{1,1}(9,:)'" : Constant  Value=[-0.80932403369743088905607919514295645058155059814453125;-0.91879672616566565590545678787748329341411590576171875;-0.5545659542950200915356617770157754421234130859375;-0.75253105915109508305960162033443339169025421142578125;0.5180007695523756172661933305789716541767120361328125;0.91741586556781129502269322983920574188232421875]
  Mux : Mux  Inputs=16
  dotprod{1..16} (16 alike) : neural/Weight Functions/dotprod
  "iz{1,1}" : Outport
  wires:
  "IW{1,1}(1,:)'"/1 -> dotprod1/1
  "pd{1,1}"/1 -> dotprod1/2, dotprod2/2, dotprod3/2, dotprod4/2, dotprod5/2, dotprod6/2, dotprod7/2, dotprod8/2, dotprod9/2, dotprod10/2, dotprod11/2, dotprod12/2, dotprod13/2, dotprod14/2, dotprod15/2, dotprod16/2
  dotprod1/1 -> Mux/1
  "IW{1,1}(2,:)'"/1 -> dotprod2/1
  dotprod2/1 -> Mux/2
  "IW{1,1}(3,:)'"/1 -> dotprod3/1
  dotprod3/1 -> Mux/3
  "IW{1,1}(4,:)'"/1 -> dotprod4/1
  dotprod4/1 -> Mux/4
  "IW{1,1}(5,:)'"/1 -> dotprod5/1
  dotprod5/1 -> Mux/5
  "IW{1,1}(6,:)'"/1 -> dotprod6/1
  dotprod6/1 -> Mux/6
  "IW{1,1}(7,:)'"/1 -> dotprod7/1
  dotprod7/1 -> Mux/7
  "IW{1,1}(8,:)'"/1 -> dotprod8/1
  dotprod8/1 -> Mux/8
  "IW{1,1}(9,:)'"/1 -> dotprod9/1
  dotprod9/1 -> Mux/9
  "IW{1,1}(10,:)'"/1 -> dotprod10/1
  dotprod10/1 -> Mux/10
  "IW{1,1}(11,:)'"/1 -> dotprod11/1
  dotprod11/1 -> Mux/11
  "IW{1,1}(12,:)'"/1 -> dotprod12/1
  dotprod12/1 -> Mux/12
  "IW{1,1}(13,:)'"/1 -> dotprod13/1
  dotprod13/1 -> Mux/13
  "IW{1,1}(14,:)'"/1 -> dotprod14/1
  dotprod14/1 -> Mux/14
  "IW{1,1}(15,:)'"/1 -> dotprod15/1
  dotprod15/1 -> Mux/15
  "IW{1,1}(16,:)'"/1 -> dotprod16/1
  dotprod16/1 -> Mux/16
  Mux/1 -> "iz{1,1}"/1
